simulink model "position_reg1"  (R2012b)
settings: Solver=ode45  StartTime=0.0  StopTime=10.0  RelTol=1e-3
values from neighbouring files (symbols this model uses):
  D = 10    [position_reg_1.m]    (also in position_reg_2.m; rad_aufhaeng_3.m = [0;ct]; rad_aufhaeng_4.m = [0;ct])
  dither_ampl = 5    [position_reg_1.m]
  fdith = 60    [position_reg_1.m]
  FG = 500    [coulomb_1.m]    (also in coulomb_10.m = 10; coulomb_11.m = 10; coulomb_2.m; coulomb_3.m)
  FH = 12    [coulomb_10.m]    (also in coulomb_11.m; coulomb_3.m = 600; coulomb_4.m = 600; position_reg_1.m = 3.956)
  I = 20    [position_reg_1.m]    (also in position_reg_2.m; suspension_1.m = 225; suspension_2.m = 225; suspension_3.m = 225)
  m = 400    [coulomb_1.m]    (also in coulomb_10.m = 10; coulomb_11.m = 10; coulomb_2.m; coulomb_3.m)
  P = 10    [position_reg_1.m]    (also in position_reg_2.m; vibration_control_1.m = em_ampl*i_ampl/2,; vibration_control_2.m = emf_ampl*i_ampl/2,; vibration_control_3.m = emf_ampl*i_ampl/2,)
  sigma_0 = 5000    [position_reg_1.m]    (also in position_reg_2.m; slip_stick_21.m = 10000; slip_stick_s_12.m = 10000; tilger_gleitreib2.m = 1000)
  sigma_1 = sqrt(sigma_0)    [position_reg_1.m]    (also in position_reg_2.m; slip_stick_21.m = sqrt(1e5); slip_stick_s_12.m = sqrt(1e5); tilger_gleitreib2.m)
  sigma_2 = 0    [position_reg_1.m]    (also in position_reg_2.m; slip_stick_21.m; slip_stick_s_12.m; tilger_gleitreib2.m)
  vs = 0.05    [position_reg_1.m]    (also in position_reg_2.m; slip_stick_21.m; slip_stick_3.m = 0.01; slip_stick_31.m)
libraries: simulink x1

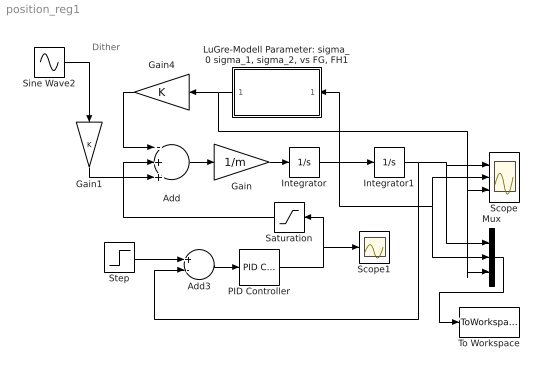
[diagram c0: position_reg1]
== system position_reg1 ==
  note: Dither
  Add : Sum  Inputs=-++
  Add3 : Sum  Inputs=+-
  Gain : Gain  Gain=1/m
  Gain1 : Gain
  Gain4 : Gain
  Integrator : Integrator
  Integrator1 : Integrator
  "LuGre-Modell Parameter: sigma_0 sigma_1, sigma_2, vs FG, FH1" : Subsystem
  Mux : Mux  Inputs=3
  PID Controller : simulink/Continuous/PID Controller  Controller=PID  TimeDomain=Continuous-time  SampleTime=1  IntegratorMethod=Forward Euler  FilterMethod=Forward Euler  Form=Parallel  P=P  I=I  D=D  N=100  InitialConditionSource=internal  InitialConditionForIntegrator=0  InitialConditionForFilter=0  ExternalReset=none  LimitOutput=off  UpperSaturationLimit=inf  LowerSaturationLimit=-inf  LinearizeAsGain=on  AntiWindupMode=none  Kb=1  TrackingMode=off  Kt=1  PParamMin=[]  PParamMax=[]  IParamMin=[]  IParamMax=[]  DParamMin=[]  DParamMax=[]  NParamMin=[]  NParamMax=[]  KbParamMin=[]  KbParamMax=[]  KtParamMin=[]  KtParamMax=[]  POutMin=[]  POutMax=[]  IOutMin=[]  IOutMax=[]  DOutMin=[]  DOutMax=[]  NOutMin=[]  NOutMax=[]  KbOutMin=[]  KbOutMax=[]  KtOutMin=[]  KtOutMax=[]  IntegratorOutMin=[]  IntegratorOutMax=[]  FilterOutMin=[]  FilterOutMax=[]  SumOutMin=[]  SumOutMax=[]  SumI1OutMin=[]  SumI1OutMax=[]  SumI2OutMin=[]  SumI2OutMax=[]  SumI3OutMin=[]  SumI3OutMax=[]  SumDOutMin=[]  SumDOutMax=[]  SaturationOutMin=[]  SaturationOutMax=[]  IntegratorContinuousStateAttributes=''  IntegratorStateMustResolveToSignalObject=off  IntegratorRTWStateStorageClass=Auto  FilterContinuousStateAttributes=''  FilterStateMustResolveToSignalObject=off  FilterRTWStateStorageClass=Auto
  Saturation : Saturate  UpperLimit=5  LowerLimit=-5  ZeroCross=off
  Scope : Scope  NumInputPorts=3
  Scope1 : Scope
  Sine Wave2 : Sin  Amplitude=dither_ampl  Frequency=fdith  SampleTime=0
  Step : Step  Time=0  SampleTime=0
  To Workspace : ToWorkspace  VariableName=y  SampleTime=-1  SaveFormat=Structure With Time
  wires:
  Add/1 -> Gain/1
  Gain/1 -> Integrator/1
  Integrator/1 -> "LuGre-Modell Parameter: sigma_0 sigma_1, sigma_2, vs FG, FH1"/1(v), Mux/2, Scope/2, Integrator1/1
  Integrator1/1 -> Add3/2, Mux/1, Scope/1
  "LuGre-Modell Parameter: sigma_0 sigma_1, sigma_2, vs FG, FH1"/1(Fr) -> Gain4/1, Scope/3, Mux/3
  Add3/1 -> PID Controller/1
  Step/1 -> Add3/1
  Gain4/1 -> Add/1
  PID Controller/1 -> Scope1/1, Saturation/1
  Saturation/1 -> Add/2
  Sine Wave2/1 -> Gain1/1
  Mux/1 -> To Workspace/1
  Gain1/1 -> Add/3

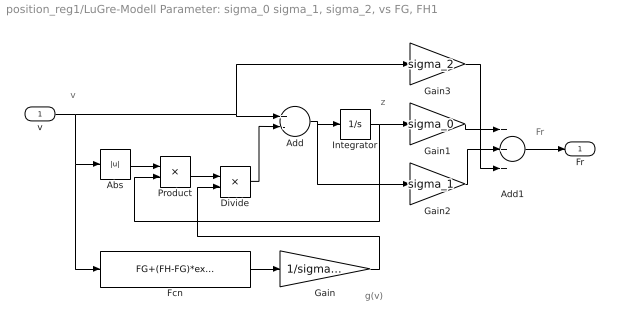
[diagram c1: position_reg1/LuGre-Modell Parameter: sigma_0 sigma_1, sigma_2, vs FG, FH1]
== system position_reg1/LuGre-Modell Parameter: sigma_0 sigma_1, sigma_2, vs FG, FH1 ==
  note: Fr
  note: v
  note: g(v)
  note: z
  v : Inport
  Abs : Abs  ZeroCross=off
  Add : Sum  Inputs=+-
  Add1 : Sum  Inputs=+++
  Divide : Product  Inputs=*/
  Fcn : Fcn  Expr=FG+(FH-FG)*exp(-(u/vs)^2)
  Gain : Gain  Gain=1/sigma_0
  Gain1 : Gain  Gain=sigma_0
  Gain2 : Gain  Gain=sigma_1
  Gain3 : Gain  Gain=sigma_2
  Integrator : Integrator  ZeroCross=off
  Product : Product
  Fr : Outport
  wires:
  v/1 -> Gain3/1, Add/1, Abs/1, Fcn/1
  Integrator/1 -> Gain1/1, Product/2
  Add/1 -> Gain2/1, Integrator/1
  Gain2/1 -> Add1/2
  Abs/1 -> Product/1
  Divide/1 -> Add/2
  Gain1/1 -> Add1/1
  Add1/1 -> Fr/1
  Gain3/1 -> Add1/3
  Fcn/1 -> Gain/1
  Gain/1 -> Divide/2
  Product/1 -> Divide/1
